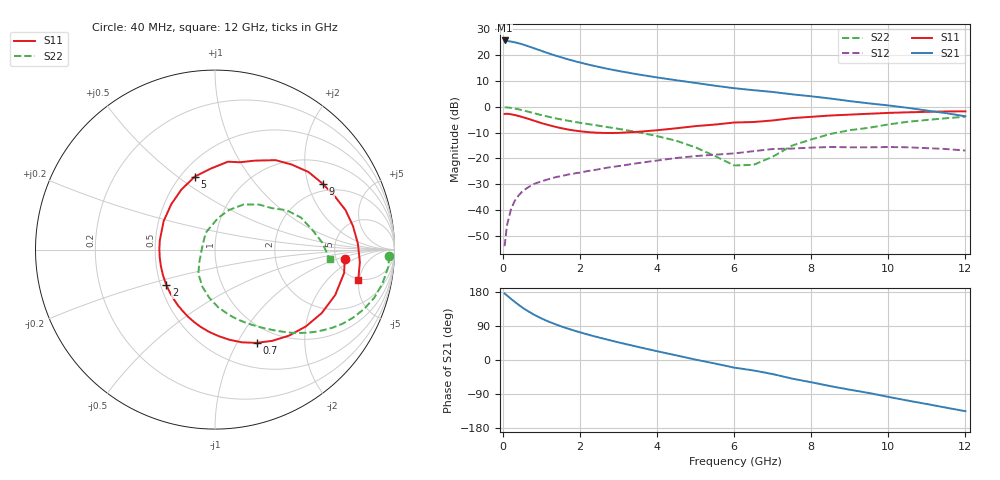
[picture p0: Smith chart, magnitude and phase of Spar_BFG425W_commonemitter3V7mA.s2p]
! Filename: 37bfg425.001
! BFG425W Field C1
! V1=8.328E-001V,V2=3.000E+000V, I1=8.713E-005A, I2=7.010E-003A
# GHz  S  MA  R 50
!  S11  S21  S12  S22
!Freq(GHz)  Mag  Ang  Mag  Ang  Mag  Ang  Mag  Ang
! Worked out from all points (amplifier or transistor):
!   44 points, 40 MHz to 12 GHz, reference 50 ohm
!   highest |S21| = 25.7 dB at 40 MHz (marker M1)
!   |S21| within 3 dB of that: start of sweep to 798.5 MHz
!   unconditionally stable (mu >= 1): 2.178 GHz to end of sweep
!   at 700 MHz: K = 0.42, MSG = 27.0 dB, |S12| = -30.8 dB
!   at 2.4 GHz: K = 1.06, MAG = 18.6 dB, |S12| = -24.4 dB
!   at 12 GHz: K = 1.44, MAG = 2.7 dB, |S12| = -17.0 dB
!   S11 on the Smith chart (normalised r, x): 40 MHz: 5.97, -1.32; 700 MHz: 0.79, -1.21; 2 GHz: 0.54, -0.24; 5 GHz: 0.59, +0.58; 9 GHz: 1.72, +2.50; 12 GHz: 4.80, -4.88
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0.04  0.725 -4.2  19.19 175.4  0.002 68.2  0.972 -2.2
0.2  0.716 -20.7  18.31 161.8  0.01 76.7  0.952 -11.5
0.3  0.692 -30.7  17.69 153.8  0.015 72.5  0.927 -16.8
0.4  0.663 -40.2  16.97 145.9  0.019 67.6  0.894 -21.7
0.5  0.632 -49.4  16.18 138.4  0.023 63.6  0.858 -26.2
0.6  0.6 -57.9  15.27 131.7  0.026 60.2  0.822 -30.2
0.7  0.569 -66.0  14.4 125.7  0.029 56.9  0.785 -33.7
0.8  0.538 -73.8  13.57 119.8  0.032 54.3  0.75 -36.9
1  0.482 -87.7  12.04 109.5  0.036 50.0  0.688 -42.3
1.3  0.419 -106.4  10.12 96.6  0.042 45.4  0.61 -49.0
1.6  0.373 -123.6  8.643 85.6  0.047 42.4  0.551 -54.4
2  0.335 -144.2  7.166 73.0  0.053 39.2  0.489 -61.1
2.2  0.323 -153.9  6.587 67.2  0.057 37.7  0.463 -64.4
3  0.312 170.4  4.926 46.5  0.071 31.3  0.373 -77.7
3.5  0.327 151.1  4.232 34.6  0.081 26.4  0.322 -86.8
4.5  0.383 119.3  3.254 12.1  0.102 14.4  0.219 -108.6
5  0.422 105.5  2.887 0.9  0.111 6.8  0.163 -124.7
6.5  0.506 74.1  2.093 -27.6  0.138 -9.8  0.075 153.3
8.5  0.677 39.7  1.441 -69.1  0.166 -46.1  0.298 57.6
9  0.704 31.3  1.286 -78.4  0.164 -54.4  0.352 45.4
10.5  0.78 9.7  0.953 -107.0  0.164 -81.5  0.511 20.5
12  0.816 -12.0  0.653 -135.1  0.142 -112.1  0.641 -4.9
